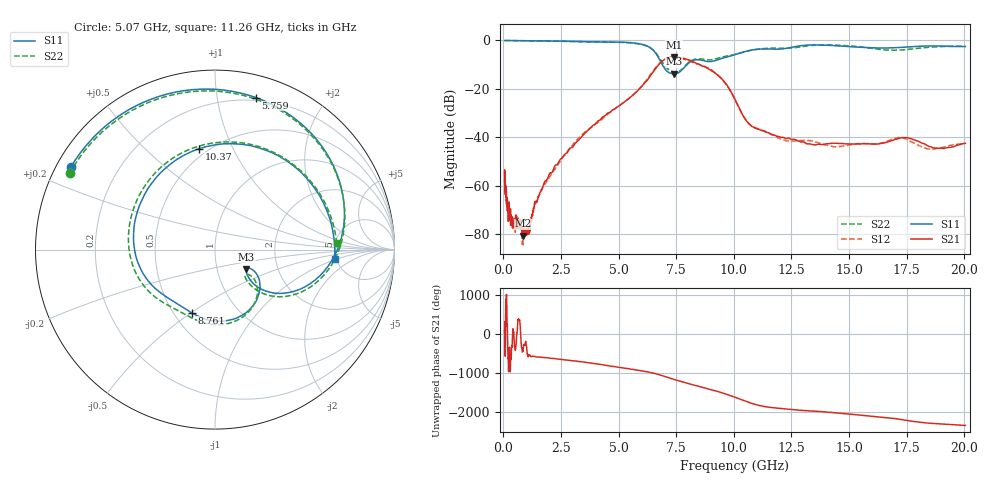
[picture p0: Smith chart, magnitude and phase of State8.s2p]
# Hz S DB R 50
!freq MagS11 AngS11 MagS21 AngS21 MagS12 AngS12 MagS22 AngS22
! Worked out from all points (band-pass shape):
!   1601 points, 50 MHz to 20.05 GHz, reference 50 ohm
!   highest |S21| = -6.84 dB at 7.402 GHz (marker M1); lowest = -80.5 dB at 865.1 MHz (marker M2)
!   |S21| within 3 dB of the highest: 6.75 GHz to 8.506 GHz (1.755 GHz wide, 23 % of centre)
!   lowest |S11| = -13.7 dB at 7.402 GHz (marker M3), VSWR 1.52, Z = 69.2 - j15.5 ohm
!   |S11| at or under -10 dB: 6.895 GHz to 7.964 GHz (1.069 GHz wide, 14.4 % of centre)
!   |S22| runs from -13.1 to 0.0 dB; largest |S21 - S12| = 0.024
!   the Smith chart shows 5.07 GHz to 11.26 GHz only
!   S11 on the Smith chart (normalised r, x): 5.07 GHz: 0.04, +0.26; 5.759 GHz: 0.18, +1.29; 8.761 GHz: 0.61, -0.50; 10.37 GHz: 0.45, +0.75; 11.26 GHz: 4.84, -0.95
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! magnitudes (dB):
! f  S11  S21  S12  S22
! 50 MHz  0.0  -55.2  -57.5  0.0
! 135.9 MHz  0.0  -66.2  -65.6  0.0
! 200.7 MHz  0.0  -69.5  -73.2  0.0
! 222.1 MHz  0.0  -74.6  -74.0  0.0
! 243.9 MHz  0.0  -67.6  -72.3  0.0
! 306.5 MHz  0.0  -75.1  -69.8  0.0
! 369.6 MHz  0.0  -74.5  -73.8  0.0
! 541.7 MHz  -0.1  -72.0  -76.9  -0.1
! 601.6 MHz  -0.1  -76.5  -73.4  -0.1
! 865.1 MHz  -0.1  -80.5  -78.5  -0.1
! 1.005 GHz  -0.1  -79.9  -80.1  -0.1
! 1.12 GHz  -0.1  -79.0  -76.7  -0.1
! 2.722 GHz  -0.3  -46.6  -46.5  -0.4
! 5.07 GHz  -0.7  -26.7  -26.5  -0.8
! 5.759 GHz  -1.1  -21.3  -21.3  -1.2
! 7.402 GHz  -13.7  -6.8  -7.1  -13.0
! 8.761 GHz  -8.5  -10.9  -10.8  -7.9
! 9.585 GHz  -7.1  -17.0  -17.1  -6.6
! 10.37 GHz  -4.9  -30.5  -30.5  -4.9
! 11.26 GHz  -3.5  -37.3  -37.1  -3.4
! 14.37 GHz  -2.1  -42.4  -43.9  -1.9
! 20.05 GHz  -2.5  -42.4  -42.4  -2.3
